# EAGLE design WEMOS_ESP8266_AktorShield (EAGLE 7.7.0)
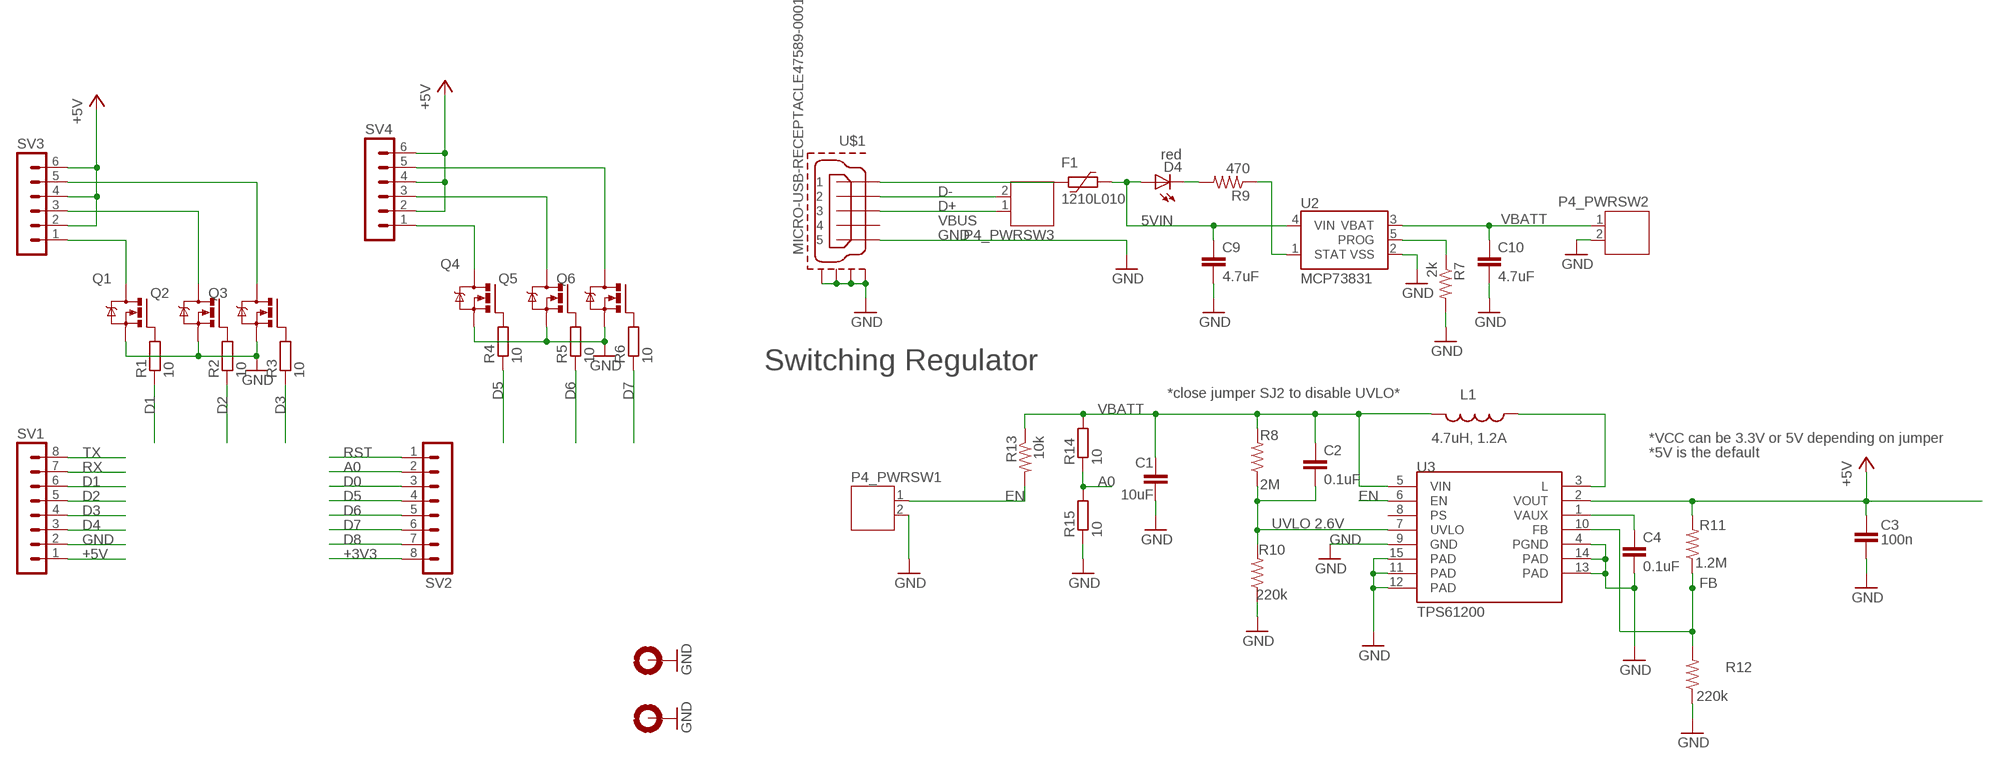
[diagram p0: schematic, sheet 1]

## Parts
C1  10uF  CAP1206  [1206]
C2  0.1uF  CAP0603-CAP  [0603-CAP]
C3  100n  CAP0805  [0805]
C4  0.1uF  CAP0603-CAP  [0603-CAP]
C9  4.7uF  CAP0603-CAP  [0603-CAP]
C10  4.7uF  CAP0603-CAP  [0603-CAP]
D4  red  LED0603  [LED-0603]
F1  1210L010  [1210L]
H7  MOUNT-PAD-ROUND3.6  [3,6-PAD]
H8  MOUNT-PAD-ROUND3.6  [3,6-PAD]
L1  4.7uH, 1.2A  INDUCTOR.  [CDRH2D09]
P4_PWRSW1  JST-PH2  [JST-PH2]
P4_PWRSW2  JST-PH2  [JST-PH2]
P4_PWRSW3  JST-PH2  [JST-PH2]
Q1  IRLML6344  [SOT23]
Q2  IRLML6344  [SOT23]
Q3  IRLML6344  [SOT23]
Q4  IRLML6344  [SOT23]
Q5  IRLML6344  [SOT23]
Q6  IRLML6344  [SOT23]
R1  10  R-EU_R0603  [R0603]
R2  10  R-EU_R0603  [R0603]
R3  10  R-EU_R0603  [R0603]
R4  10  R-EU_R0603  [R0603]
R5  10  R-EU_R0603  [R0603]
R6  10  R-EU_R0603  [R0603]
R7  2k  RESISTOR0603-RES  [0603-RES]
R8  2M  RESISTOR0603-RES  [0603-RES]
R9  470  RESISTOR0603-RES  [0603-RES]
R10  220k  RESISTOR0603-RES  [0603-RES]
R11  1.2M  RESISTOR0603-RES  [0603-RES]
R12  220k  RESISTOR0603-RES  [0603-RES]
R13  10k  RESISTOR0603-RES  [0603-RES]
R14  10  R-EU_R0603  [R0603]
R15  10  R-EU_R0603  [R0603]
SV1  MA08-1SMALL  [MA08-1S]
SV2  MA08-1SMALL  [MA08-1S]
SV3  MA06-1  [MA06-1]
SV4  MA06-1  [MA06-1]
U2  MCP73831  [SOT23-5]
U3  TPS61200  [QFN-10_PAD]
U$1  MICRO-USB-RECEPTACLE47589-0001  [47589-0001]

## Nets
5VIN: C9.1 D4.A F1.1 U2.4(VIN)
+3V3: SV2.8
+5V: C3.1 R11.2 SV1.1 SV3.2 SV3.4 SV3.6 SV4.2 SV4.4 SV4.6 U3.2(VOUT)
A0: R14.1 R15.2 SV2.2
D0: SV2.3
D1: R1.1 SV1.6
D2: R2.1 SV1.5
D3: R3.1 SV1.4
D4: SV1.3
D5: R4.1 SV2.4
D6: R5.1 SV2.5
D7: R6.1 SV2.6
D8: SV2.7
D+: P4_PWRSW3.1 U$1.3
D-: P4_PWRSW3.2 U$1.2
EN: P4_PWRSW1.1 R13.2 U3.6(EN)
FB: R11.1 R12.2 U3.10(FB)
GND: C1.2 C3.2 C4.2 C9.2 C10.2 H7.B3,6(MOUNT) H8.B3,6(MOUNT) P4_PWRSW1.2 P4_PWRSW2.2 Q1.2(S) Q2.2(S) Q3.2(S) Q4.2(S) Q5.2(S) Q6.2(S) R7.2 R10.1 R12.1 R15.1 SV1.2 U2.2(VSS) U3.4(PGND) U3.9(GND) U3.11(PAD) U3.12(PAD) U3.13(PAD) U3.14(PAD) U3.15(PAD) U$1.5 U$1.CASING1(GND1) U$1.CASING2(GND2) U$1.CASING3(GND3) U$1.CASING4(GND4)
N$1: Q1.1(G) R1.2
N$2: Q2.1(G) R2.2
N$3: Q3.1(G) R3.2
N$4: Q3.3(D) SV3.5
N$5: Q1.3(D) SV3.1
N$6: Q2.3(D) SV3.3
N$7: Q4.1(G) R4.2
N$8: Q5.1(G) R5.2
N$9: Q6.1(G) R6.2
N$10: Q4.3(D) SV4.1
N$11: Q5.3(D) SV4.3
N$12: Q6.3(D) SV4.5
N$13: R7.1 U2.5(PROG)
N$14: R9.1 U2.1(STAT)
N$15: D4.C R9.2
N$16: L1.P$1 U3.3(L)
N$17: C4.1 U3.1(VAUX)
RST: SV2.1
RX: SV1.7
TX: SV1.8
UVLO: C2.2 R8.1 R10.2 U3.7(UVLO)
VBATT: C1.1 C2.1 C10.1 L1.P$2 P4_PWRSW2.1 R8.2 R13.1 R14.2 U2.3(VBAT) U3.5(VIN)
VBUS: F1.2 U$1.1
Unconnected: U3.8(PS) U$1.4

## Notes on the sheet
- Switching Regulator
- *close jumper SJ2 to disable UVLO*
- *VCC can be 3.3V or 5V depending on jumper
- *5V is the default
- UVLO 2.6V

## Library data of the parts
C1 = CH_passive:CAP: Capacitor; MF: KEMET; MPN: C1206C106K8RACTU; OC_FARNELL: 1288264
C2 C4 = SparkFun:CAP: Capacitor; MF: YAGEO (PHYCOMP); MPN: CC0603MRY5V9BB104; OC_FARNELL: 431989
C3 = CH_passive:CAP: Capacitor; MF: YAGEO (PHYCOMP); MPN: CC0603MRY5V9BB104; OC_FARNELL: 431989
C9 C10 = SparkFun:CAP: Capacitor; MF: KEMET; MPN: C0603C475K8PACTU; OC_FARNELL: 1572625
D4 = SparkFun:LED: LEDs; MF: OSRAM; MPN: LSQ976-Z; OC_FARNELL: 1226390
F1 = polyfuse-smd_10:?: Polyfuse Resettable PTC; MF: LITTELFUSE; MPN: 1210L010WR; OC_FARNELL: 1822206; OC_NEWARK: 18M4781
H7 H8 = holes_new:MOUNT-PAD-ROUND: MOUNTING PAD, round; OC_FARNELL: unknown
L1 = SparkFun:INDUCTOR: Inductors; MF: MURATA; MPN: LQH3NPN4R7MJ0L; OC_FARNELL: 2219271
P4_PWRSW1-P4_PWRSW3 = jst-ph:JST-PH2; MF: JST (JAPAN SOLDERLESS TERMINALS); MPN: B2B-PH-K-S(LF)(SN); OC_FARNELL: 9491856
Q1-Q6 = myDBv7:IRLML6344; MF: INFINEON; MPN: IRLML6344TRPBF; OC_FARNELL: 1857299
R1-R6 R14 R15 = rcl:R-EU_: RESISTOR, European symbol; MF: VISHAY; MPN: CRCW060310R0FKEA; OC_FARNELL: 1469751
R7 = SparkFun:RESISTOR: Resistor; MF: YAGEO (PHYCOMP); MPN: RC0603FR-072K2L.; OC_FARNELL: 9238522
R8 = SparkFun:RESISTOR: Resistor; MF: KOA SPEER ELECTRONICS; MPN: RK73H1JTTD1204F; OC_FARNELL: 1811595
R9 = SparkFun:RESISTOR: Resistor; MF: MULTICOMP; MPN: MCHP03W8F4700T5E; OC_FARNELL: 1576273
R10 R12 = SparkFun:RESISTOR: Resistor; MF: MULTICOMP; MPN: MCHP03W8F2203T5E; OC_FARNELL: 1576314
R11 = SparkFun:RESISTOR: Resistor; MF: MULTICOMP; MPN: MCMR06W2004FTL; OC_FARNELL: 2073340
R13 = SparkFun:RESISTOR: Resistor; MF: MULTICOMP; MPN: MCMR06X1002FTL; OC_FARNELL: 2073349
SV1 SV2 = con-pin-header:MA08-1: PIN HEADER; OC_FARNELL: unknown
SV3 SV4 = con-pin-header:MA06-1: PIN HEADER; OC_FARNELL: unknown
U2 = SparkFun:MCP73831: Microchip's MCP73831 Miniature single cell, fully integrated Li-Ion, Li-polymer charge management controller http://ww1.microchip.com/downloads/en/DeviceDoc/21984a.pdf; MF: MICROCHIP; MPN: MCP73831T-2ACI/OT; OC_FARNELL: 1332158
U3 = SparkFun:TPS61200: DC to DC Booster; MF: TEXAS INSTRUMENTS; MPN: TPS61200DRCT; OC_FARNELL: 1471238
U$1 = con-molex-usb:MICRO-USB-RECEPTACLE: MICRO USB RECEPTACLES Micro-USB Receptacles, SMT, Lead-Free from MOLEX. (C) 2014 Tomasz Boleslaw CEDRO, cederom@tlen.pl, http://www.tomek.cedro.info. Version 0.1 (2014-01-17): Initial release. Version 0.2 (2014-02-06): Updated 47589-0001 footprint pins/pads/milling. Following devices are included: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; MF: MOLEX; MPN: 47589-0001; OC_FARNELL: 1568023

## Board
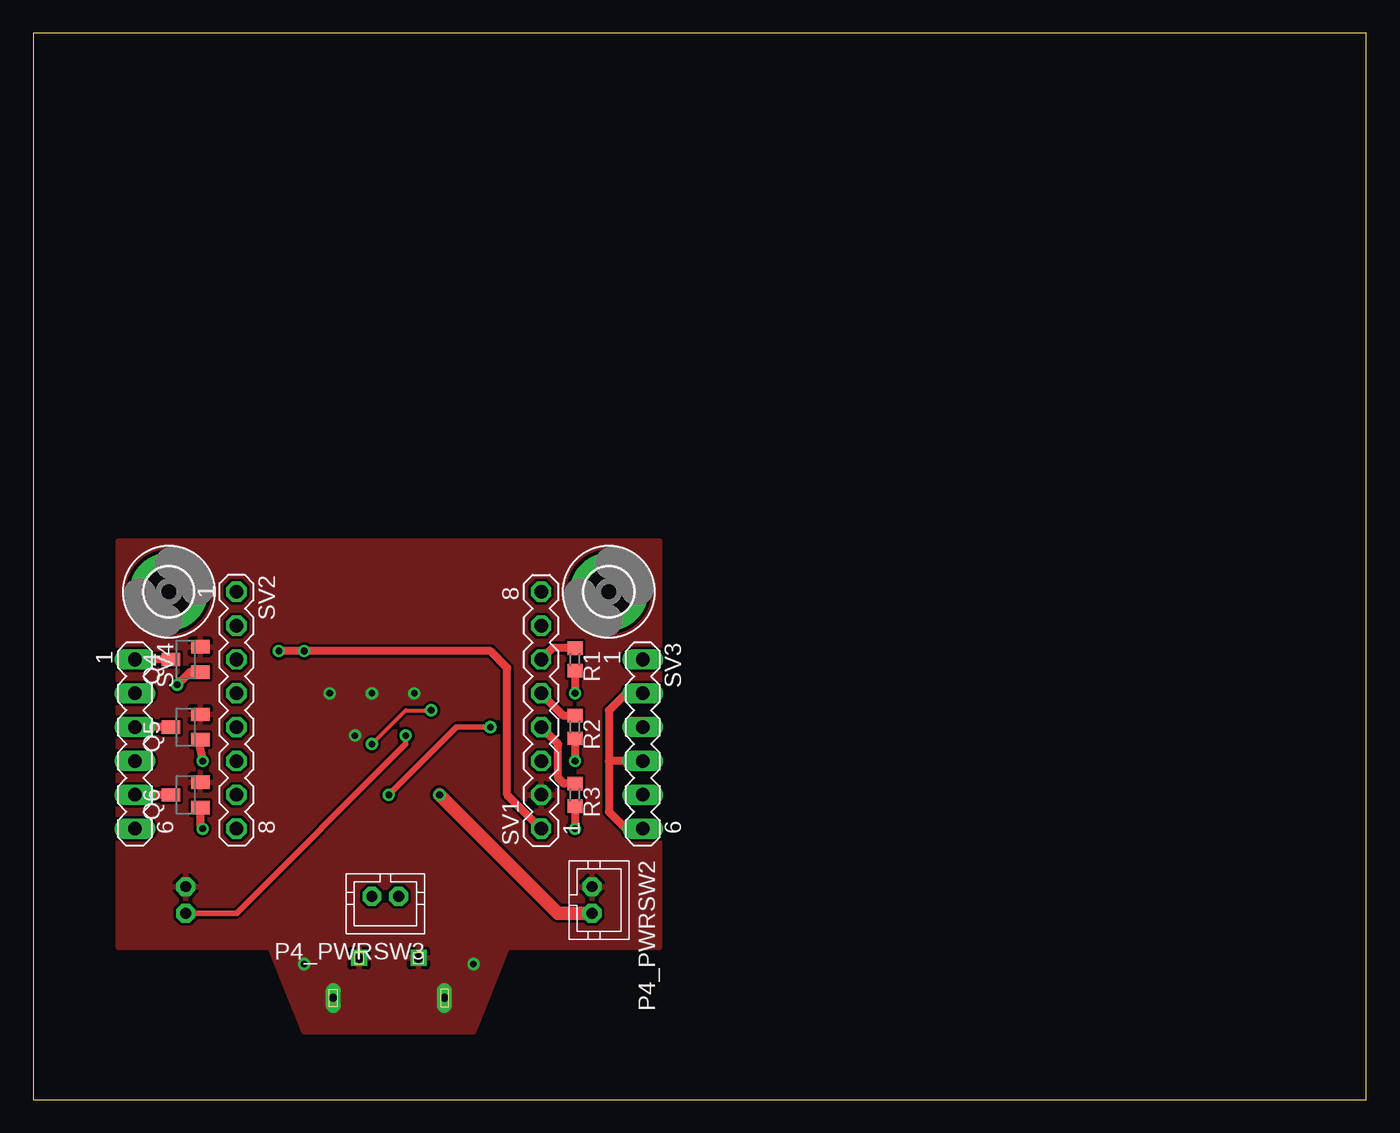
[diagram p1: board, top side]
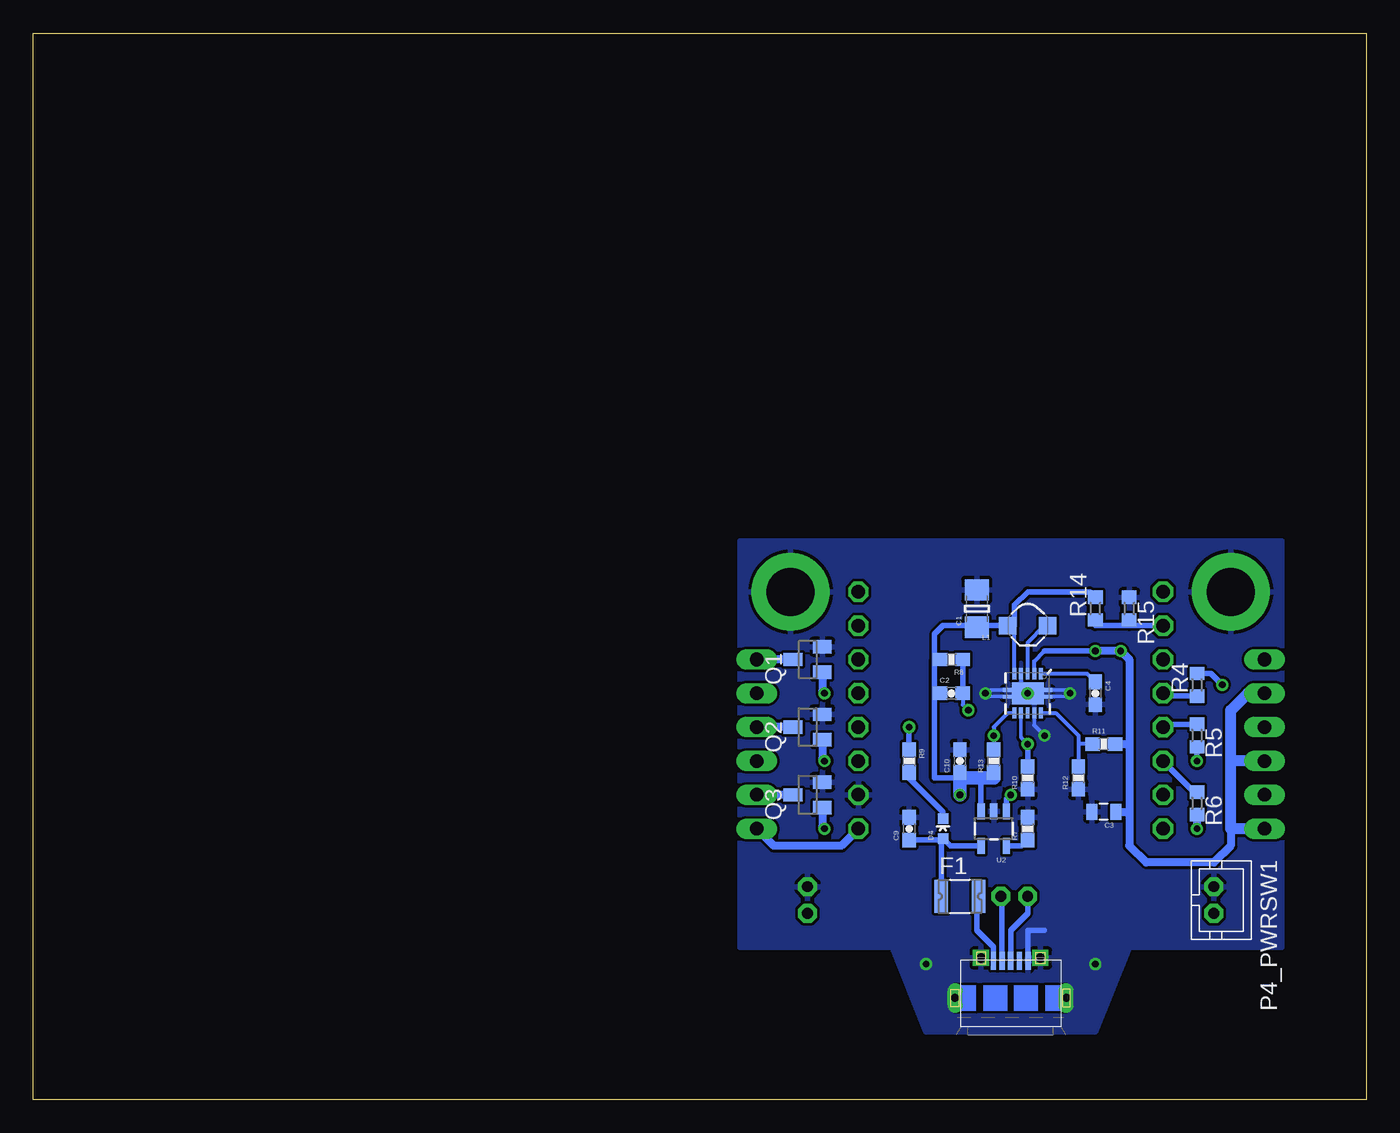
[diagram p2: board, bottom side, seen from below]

Size 100 x 80 mm. Coordinates in mm from the lower left corner, seen from the top.
Outline: 0,0 100,0 100,80 0,80 0,0
Copper layers (1*16): Top 0.035mm / dielectric 1.5mm / Bottom 0.035mm
Design rules "default": minimum track width 10mil, minimum drill 0.6mm, track to track 8mil, track to pad 8mil, pad to pad 8mil, via to via 8mil, smd to smd 8mil, copper to edge 40mil, drill to drill 8mil, minimum pad ring 10mil, minimum via ring 8mil, stop-mask expansion 4mil, vias tented up to drill 0mil, thermal gap 10mil

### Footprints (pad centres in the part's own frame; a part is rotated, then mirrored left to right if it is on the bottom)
1206 = smd 1.6 x 1.8: 1 -1.4,0; 2 1.4,0
0603-CAP = smd 1.1 x 1: 1 -0.85,0; 2 0.85,0
0805 = smd 0.8 x 1.2: 1 -0.9,0; 2 0.9,0
LED-0603 = smd 0.8 x 0.8: A 0,-0.75; C 0,0.75
1210L = smd 1 x 2.5: 1 -1.4,0; 2 1.4,0
3,6-PAD = drill 3.6 pad 5.842: B3,6 0,0
CDRH2D09 = smd 1.3 x 1.3: P$1 -1.5,0; P$2 1.5,0
JST-PH2 = drill 0.813 pad 1.422 octagon: 1 0,0; 2 -2,0
SOT23 = smd 1 x 1.4: 1 -0.95,-1.1; 2 0.95,-1.1; 3 0,1.1
R0603 = smd 1 x 1.1: 1 -0.85,0; 2 0.85,0
0603-RES = smd 1.1 x 1: 1 -0.85,0; 2 0.85,0
MA08-1S = drill 1.016 octagon: 1 -8.89,0; 2 -6.35,0; 3 -3.81,0; 4 -1.27,0; 5 1.27,0; 6 3.81,0; 7 6.35,0; 8 8.89,0
MA06-1 = drill 1.016 long: 1 -6.35,0; 2 -3.81,0; 3 -1.27,0; 4 1.27,0; 5 3.81,0; 6 6.35,0
SOT23-5 = smd 0.55 x 1.2: 1 -0.95,-1.3; 2 0,-1.3; 3 0.95,-1.3; 4 0.95,1.3; 5 -0.95,1.3
QFN-10_PAD = smd 0.297 x 0.85: 1 -1,-1.475; 2 -0.5,-1.475; 3 0,-1.475; 4 0.5,-1.475; 5 1,-1.475; 6 1,1.475; 7 0.5,1.475; 8 0,1.475; 9 -0.5,1.475; 10 -1,1.475 | smd 0.7 x 0.28: 11 -1.5,0.25; 12 -1.5,-0.25; 13 1.5,0.25; 14 1.5,-0.25 | smd 2.4 x 1.65: 15 0,0
47589-0001 = smd 1.35 x 0.4: 1 2.8,1.3; 2 2.8,0.65; 3 2.8,0; 4 2.8,-0.65; 5 2.8,-1.3 | drill 0.6 pad 0.95 long: CASING1 0,4.175; CASING2 0,-4.175 | drill 0.7 pad 1.1 square: CASING3 3,2.225; CASING4 3,-2.225

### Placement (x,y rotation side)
C1  29.21,36.83 90 bottom
C2  31.11,30.48 0 bottom
C3  19.68,21.59 180 bottom
C4  20.32,30.48 270 bottom
C9  34.29,20.32 90 bottom
C10  30.48,25.4 90 bottom
D4  31.75,20.32 0 bottom
F1  30.48,15.24 0 bottom
H7  10.16,38.1 0 top
H8  43.18,38.1 0 top
L1  25.4,35.56 180 bottom
P4_PWRSW1  11.43,13.97 270 bottom
P4_PWRSW2  41.91,13.97 270 top
P4_PWRSW3  25.4,15.24 180 top
Q1  41.91,33.02 90 bottom
Q2  41.91,27.94 90 bottom
Q3  41.91,22.86 90 bottom
Q4  11.43,33.02 90 top
Q5  11.43,27.94 90 top
Q6  11.43,22.86 90 top
R1  40.64,33.02 270 top
R2  40.64,27.94 270 top
R3  40.64,22.86 270 top
R4  12.7,31.11 90 bottom
R5  12.7,27.3 270 bottom
R6  12.7,22.23 270 bottom
R7  25.4,20.32 90 bottom
R8  31.11,33.02 180 bottom
R9  34.29,25.4 270 bottom
R10  25.4,24.13 90 bottom
R11  19.68,26.67 0 bottom
R12  21.59,24.13 90 bottom
R13  27.94,25.4 90 bottom
R14  20.32,36.83 90 bottom
R15  17.78,36.83 270 bottom
SV1  38.1,29.21 90 top
SV2  15.24,29.21 270 top
SV3  45.72,26.67 270 top
SV4  7.62,26.67 270 top
U2  27.94,20.32 180 bottom
U3  25.4,30.48 180 bottom
U$1  26.67,7.62 90 bottom

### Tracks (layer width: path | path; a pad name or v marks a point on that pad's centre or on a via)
5VIN
  Bottom 0.406: U2.4 31.2,19.02 D4.A | C9.1 31.85,19.47 D4.A | F1.1 31.88,19.44 D4.A
+5V  (via drill 0.5)
  Top 0.61: SV3.2 44.45,30.48 43.18,29.21 43.18,25.4 | SV3.4 43.18,25.4 | 43.18,25.4 43.18,21.59 44.45,20.32 SV3.6 | SV1.1 35.56,22.86 35.56,32.38 34.29,33.66 v20.32,33.66 v18.41,33.66
  Bottom 0.305: U3.2 24.9,32.88 24.13,33.66
  Bottom 0.406: 24.13,33.66 v20.32,33.66
  Bottom 0.61: SV1.1 39.37,19.05 44.45,19.05 SV3.6 | 10.16,20.32 10.16,19.05 11.43,17.78 16.51,17.78 17.78,19.05 17.78,21.59 | 17.78,26.67 17.78,33.02 v18.41,33.66 v20.32,33.66 | 17.78,26.67 17.78,21.59 | R11.2 17.78,26.67 | C3.1 17.78,21.59
  Bottom 0.813: SV4.6 10.16,20.32 10.16,25.4 | 10.16,25.4 10.16,29.21 8.89,30.48 SV4.2 | SV4.4 10.16,25.4
A0
  Bottom 0.406: SV2.2 17.78,35.56 | 17.78,35.56 20.32,35.56 R14.1 | R15.2 17.78,35.56
D1
  Top 0.61: R1.1 38.95,33.87 SV1.6
D2
  Top 0.61: R2.1 39.79,28.79 SV1.5
D3
  Top 0.61: R3.1 39.79,23.71 39.37,24.13 39.37,26.67 SV1.4
D5
  Bottom 0.406: R4.1 15.03,30.27 SV2.4
D6
  Bottom 0.406: R5.1 15.03,28.16 SV2.5
D7
  Bottom 0.406: R6.1 12.91,23.07 SV2.6
D+
  Bottom 0.406: P4_PWRSW3.1 25.4,13.97 26.67,12.7 U$1.3
D-
  Bottom 0.406: U$1.2 27.32,15.16 P4_PWRSW3.2
EN  (via drill 0.5)
  Top 0.406: P4_PWRSW1.1 15.24,13.97 27.94,26.67 v27.94,27.3
  Bottom 0.254: U3.6 26.88,29
  Bottom 0.305: 26.88,29 27.94,27.94 v27.94,27.3 R13.2
FB
  Bottom 0.305: U3.10 23.29,29 21.59,27.3 21.59,26.67 | 21.59,26.67 R12.2 | R11.1 21.59,26.67
GND  (via drill 0.5)
  Bottom 0.254: U3.9 24.9,28.07 | U3.13 28.32,30.23 v28.57,30.48 28.32,30.73 U3.14 | U3.11 22.48,30.23 v22.23,30.48 22.48,30.73 U3.12
  Bottom 0.305: 24.9,28.07 v24.13,27.3 | U3.4 25.9,30.98 U3.15 25.15,30.73 U3.12
  Bottom 0.406: U$1.5 25.37,12.67 25.4,12.7 24.13,12.7
  other vias: 25.4,30.48 20.32,10.16 33.02,10.16
  pour Top: 6.35,41.91 46.99,41.91 46.99,11.43 35.56,11.43 33.02,5.08 20.32,5.08 17.78,11.43 6.35,11.43
  pour Bottom: 6.35,41.91 46.99,41.91 46.99,11.43 35.56,11.43 33.02,5.08 20.32,5.08 17.78,11.43 6.35,11.43
N$1  (via drill 0.5)
  Top 0.61: R1.2 v40.64,30.48
  Bottom 0.61: Q1.1 40.81,30.65 v40.64,30.48
N$2  (via drill 0.5)
  Top 0.61: R2.2 v40.64,25.4
  Bottom 0.61: Q2.1 40.81,25.57 v40.64,25.4
N$3  (via drill 0.5)
  Top 0.61: R3.2 v40.64,20.32
  Bottom 0.61: Q3.1 40.81,20.49 v40.64,20.32
N$4
  Bottom 0.61: Q3.3 SV3.5
N$5
  Bottom 0.61: Q1.3 SV3.1
N$6
  Bottom 0.61: Q2.3 SV3.3
N$7  (via drill 0.5)
  Top 0.61: Q4.1 11.75,32.07 v10.79,31.11
  Bottom 0.406: R4.2 11.64,31.96 v10.79,31.11
N$8  (via drill 0.5)
  Top 0.61: Q5.1 12.38,26.99 v12.7,25.4
  Bottom 0.406: R5.2 v12.7,25.4
N$9  (via drill 0.5)
  Top 0.61: Q6.1 12.53,20.49 v12.7,20.32
  Bottom 0.61: R6.2 v12.7,20.32
N$10
  Top 0.61: Q4.3 SV4.1
N$11
  Top 0.61: Q5.3 SV4.3
N$12
  Top 0.61: Q6.3 SV4.5
N$13
  Bottom 0.406: U2.5 25.85,19.02 R7.1
N$14  (via drill 0.5)
  Top 0.406: v34.29,27.94 31.75,27.94 v26.67,22.86
  Bottom 0.406: U2.1 26.99,22.54 v26.67,22.86 | R9.1 v34.29,27.94
N$15
  Bottom 0.406: D4.C 31.75,21.59 34.29,24.13 R9.2
N$16
  Bottom 0.305: U3.3 25.4,34.29 24.13,35.56 24.13,35.33 L1.P$1
N$17
  Bottom 0.305: U3.1 20.95,31.95 C4.1
UVLO  (via drill 0.5)
  Top 0.305: v25.4,26.67 27.94,29.21 v29.84,29.21
  Bottom 0.254: U3.7 25.9,27.17
  Bottom 0.305: 25.9,27.17 v25.4,26.67 | C2.2 30.27,29.63 v29.84,29.21
  Bottom 0.406: R10.2 v25.4,26.67 | R8.1 C2.2
VBATT  (via drill 0.5)
  Top 1.016: P4_PWRSW2.1 39.37,13.97 v30.48,22.86
  Bottom 0.305: U3.5 26.4,35.56
  Bottom 0.406: U2.3 28.89,23.81 29.21,24.13 | R13.1 27.94,24.13 | 30.48,24.13 32.38,24.13 32.38,30.48 | 32.38,30.48 32.38,33.02 | L1.P$2 31.75,35.56 32.38,34.92 32.38,33.02 | 32.38,33.02 R8.2 31.75,33.02 | C1.1 29.21,35.56 L1.P$2 | L1.P$2 26.67,35.56 26.8,35.66 | 26.8,35.66 L1.P$2 | C2.1 32.38,30.48 | R14.2 20.74,38.1 25.4,38.1 26.4,37.1 26.4,35.56 26.5,35.66 26.8,35.66
  Bottom 1.016: 27.94,24.13 29.21,24.13 30.48,24.13 | C10.1 30.48,24.13 | 30.48,24.13 v30.48,22.86
VBUS
  Bottom 0.406: F1.2 29.21,15.11 29.21,12.7 27.97,11.46 U$1.1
